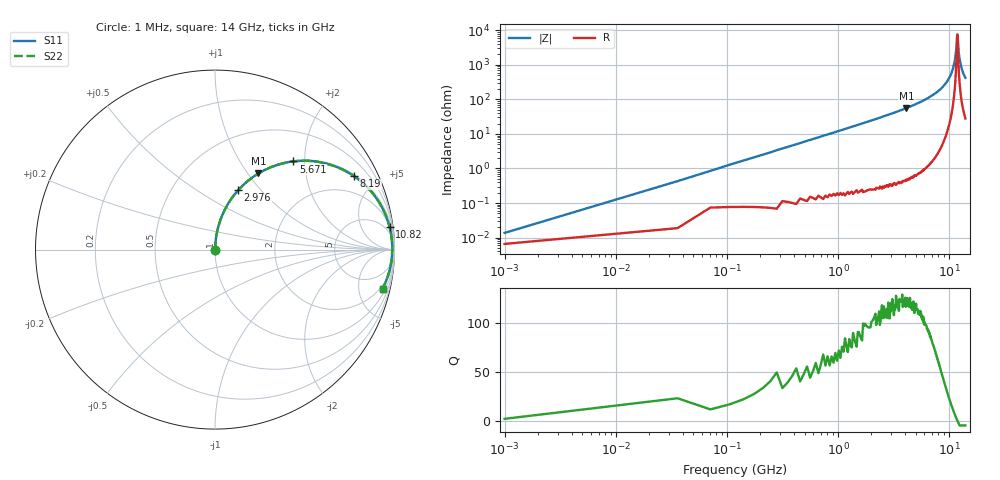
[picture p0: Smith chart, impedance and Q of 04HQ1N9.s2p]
! Coilcraft 0403HQ-1N9 Chip Inductor
! 13 February 2004
# MHZ S MA R 50
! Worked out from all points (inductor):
!   401 points, 1 MHz to 14 GHz, reference 50 ohm
!   read as one part in series: L = 1.91 nH near 71 MHz
!   highest Q = 123 at 4.131 GHz (marker M1), where L = 2.16 nH
!   self-resonance near 11.83 GHz
!   S11 on the Smith chart (normalised r, x): 1 MHz: 1.00, +0.00; 2.976 GHz: 1.01, +0.76; 5.671 GHz: 1.02, +1.76; 8.19 GHz: 1.06, +3.75; 10.82 GHz: 2, +15; 14 GHz: 1.55, -8.40
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1  0.0001769 42.4  1 -0.0  1 -0.0  0.0001769 42.4
105.992  0.013 86.6  0.999 -0.7  0.999 -0.7  0.013 86.6
210.985  0.025 86.7  0.999 -1.4  0.999 -1.4  0.025 86.7
385.972  0.046 86.0  0.998 -2.6  0.998 -2.6  0.046 86.0
665.952  0.079 84.4  0.995 -4.6  0.995 -4.6  0.079 84.4
1085.922  0.129 81.8  0.99 -7.4  0.99 -7.4  0.129 81.8
2345.832  0.279 73.2  0.958 -16.2  0.958 -16.2  0.279 73.2
2975.787  0.354 68.8  0.932 -20.7  0.932 -20.7  0.354 68.8
4130.705  0.488 60.3  0.869 -29.2  0.869 -29.2  0.488 60.3
4690.665  0.551 56.1  0.83 -33.4  0.83 -33.4  0.551 56.1
5670.595  0.657 48.4  0.748 -41.1  0.748 -41.1  0.657 48.4
7000.5  0.784 37.6  0.611 -51.7  0.611 -51.7  0.784 37.6
8190.415  0.876 27.9  0.468 -61.1  0.468 -61.1  0.876 27.9
9345.333  0.939 18.5  0.318 -69.8  0.318 -69.8  0.939 18.5
10815.23  0.981 7.3  0.127 -77.7  0.127 -77.7  0.981 7.3
11340.19  0.986 3.5  0.062 -75.6  0.062 -75.6  0.986 3.5
11690.17  0.988 1.1  0.022 -55.7  0.022 -55.7  0.988 1.1
11865.15  0.988 -0.1  0.013 9.5  0.013 9.5  0.988 -0.1
12215.13  0.986 -2.4  0.045 70.8  0.045 70.8  0.986 -2.4
12565.1  0.983 -4.7  0.083 76.1  0.083 76.1  0.983 -4.7
13160.06  0.975 -8.3  0.146 76.1  0.146 76.1  0.975 -8.3
14000  0.959 -13.1  0.228 73.0  0.228 73.0  0.959 -13.1
